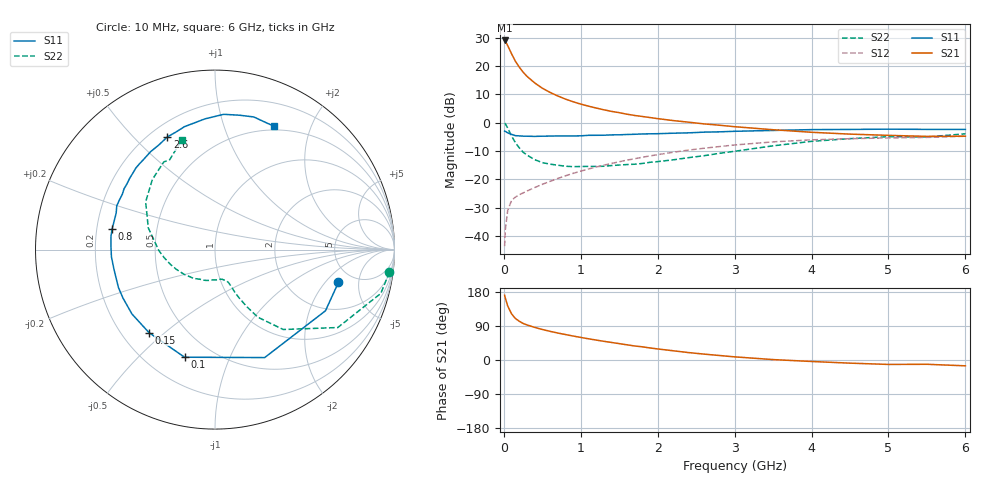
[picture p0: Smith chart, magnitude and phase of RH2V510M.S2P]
! SIEMENS Small Signal Semiconductors
! BFR106
! Si NPN RF Bipolar Junction Transistor in SOT23
! VCE = 2.5 V  IC = 10 mA
! Common Emitter S-Parameters:  August  1996
# GHz  S  MA  R  50
!  f  S11  S21  S12  S22
! GHz  MAG  ANG  MAG  ANG  MAG  ANG  MAG  ANG
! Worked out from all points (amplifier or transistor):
!   36 points, 10 MHz to 6 GHz, reference 50 ohm
!   highest |S21| = 29.1 dB at 10 MHz (marker M1)
!   |S21| within 3 dB of that: start of sweep to 70.86 MHz
!   unconditionally stable (mu >= 1): 475.5 MHz to 2.241 GHz; 4.93 GHz to end of sweep
!   at 250 MHz: K = 0.72, MSG = 21.3 dB, |S12| = -24.8 dB
!   at 1.4 GHz: K = 1.10, MAG = 7.2 dB, |S12| = -14.4 dB
!   at 6 GHz: K = 1.02, MAG = -0.8 dB, |S12| = -4.8 dB
!   S11 on the Smith chart (normalised r, x): 10 MHz: 3.77, -2.79; 100 MHz: 0.35, -0.69; 150 MHz: 0.31, -0.44; 800 MHz: 0.26, +0.09; 2.6 GHz: 0.27, +0.63; 6 GHz: 0.46, +1.49
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0.01  0.7117 -14.9  28.39 170.8  0.0066 84.8  0.9801 -7.4
0.02  0.7035 -29.0  27.57 163.2  0.0131 75.9  0.9555 -14.8
0.05  0.6622 -65.3  23.08 142.7  0.0282 61.7  0.8103 -32.4
0.1  0.6231 -105.8  16.57 121.9  0.0423 48.9  0.5856 -49.5
0.15  0.5909 -128.5  12.2 109.6  0.0486 44.7  0.4449 -57.7
0.2  0.5855 -142.2  9.628 102.3  0.0534 44.8  0.3609 -61.0
0.25  0.5795 -152.2  7.84 96.5  0.0575 45.3  0.3021 -63.4
0.3  0.578 -158.6  6.614 92.6  0.0621 47.7  0.269 -64.9
0.4  0.5735 -169.0  5.058 86.1  0.0715 50.6  0.2228 -66.3
0.5  0.5784 -176.0  4.072 80.6  0.0816 53.9  0.1976 -67.8
0.6  0.5805 177.7  3.436 75.7  0.0921 55.8  0.1854 -69.9
0.7  0.5843 172.6  2.973 71.2  0.1035 57.5  0.1778 -73.1
0.8  0.5846 168.8  2.617 67.2  0.1153 58.4  0.1705 -76.2
1.1  0.5994 155.9  1.962 56.0  0.1523 59.6  0.1691 -88.0
1.3  0.6012 149.2  1.692 49.3  0.1781 59.0  0.1703 -96.8
1.6  0.6196 140.1  1.415 40.1  0.2181 57.2  0.1824 -111.5
2.2  0.6528 123.4  1.092 24.4  0.3008 50.6  0.2209 -141.6
2.6  0.6817 112.9  0.954 15.6  0.3539 44.8  0.2611 -161.4
3.5  0.7305 94.4  0.752 1.1  0.4592 30.1  0.3907 162.0
4.5  0.7611 79.6  0.629 -8.3  0.5223 13.5  0.5236 131.8
5.5  0.7623 68.0  0.574 -11.3  0.5505 3.0  0.5606 116.8
6  0.7618 64.3  0.578 -15.4  0.5773 -4.4  0.6368 107.0
